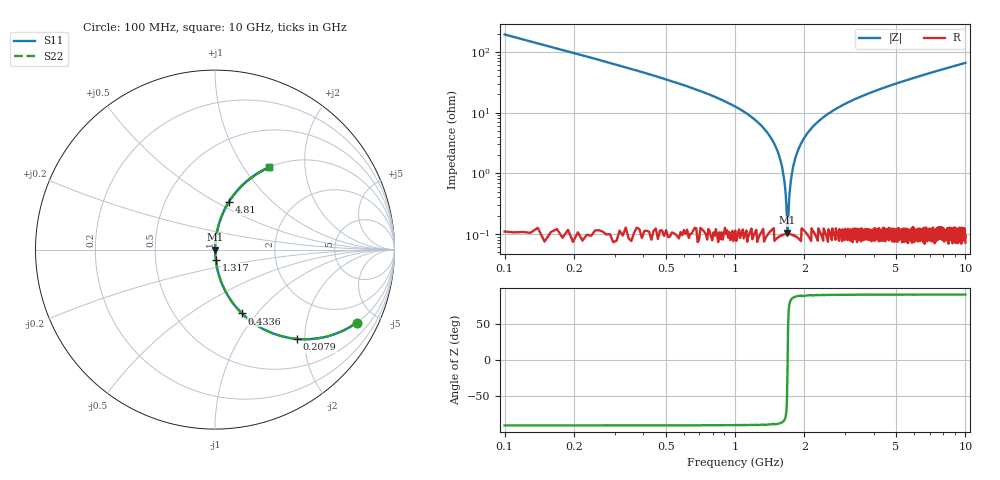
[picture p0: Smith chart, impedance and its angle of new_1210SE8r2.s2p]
!	AVX	Thin	Film	Operation	Date:	April 2007
!	Description:	Accu-P®	"Series,"	Thin	"Film,"	"SMD,"	RF	Capacitor
!	Part	Number:	12101J8R2BBT
!	100	MHz	-	5.05	GHz
!	Serial	Measurements
#	MHZ	S	MA	R	50
!	S11	S21	S12	S22
!	dB	Phase	dB	Phase	dB	Phase	dB	Phase
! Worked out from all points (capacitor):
!   1010 points, 100 MHz to 10 GHz, reference 50 ohm
!   read as one part in series: C = 8.2 pF near 149.1 MHz
!   lowest |Z| = 105 mohm at 1.689 GHz (marker M1)
!   series resonance near 1.692 GHz, so ESL is about 1.1 nH
!   S11 on the Smith chart (normalised r, x): 100 MHz: 1.00, -3.87; 207.9 MHz: 1.00, -1.84; 433.6 MHz: 1.00, -0.84; 1.317 GHz: 1.00, -0.12; 4.81 GHz: 1.00, +0.57; 10 GHz: 1.00, +1.32
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100  0.888 -27.3  0.459 62.6  0.459 62.6  0.888 -27.3
207.929  0.676 -47.4  0.736 42.6  0.736 42.6  0.676 -47.4
433.598  0.386 -67.2  0.922 22.7  0.922 22.7  0.386 -67.2
737.76  0.208 -77.7  0.977 12.0  0.977 12.0  0.208 -77.7
1316.65  0.058 -85.7  0.997 3.3  0.997 3.3  0.058 -85.7
1463.826  0.033 -86.4  0.998 1.9  0.998 1.9  0.033 -86.4
1552.131  0.02 -86.0  0.999 1.1  0.999 1.1  0.02 -86.0
1611.001  0.011 -84.3  0.999 0.6  0.999 0.6  0.011 -84.3
1660.059  0.00446 -76.8  0.999 0.2  0.999 0.2  0.00446 -76.8
1689.495  0.00105 -17.5  0.999 0.0  0.999 0.0  0.00105 -17.5
1728.741  0.00505 78.3  0.999 -0.3  0.999 -0.3  0.00505 78.3
1758.176  0.00888 83.0  0.999 -0.5  0.999 -0.5  0.00888 83.0
1817.047  0.016 85.6  0.999 -0.9  0.999 -0.9  0.016 85.6
1895.54  0.026 86.3  0.999 -1.5  0.999 -1.5  0.026 86.3
2189.891  0.06 85.6  0.997 -3.4  0.997 -3.4  0.06 85.6
2670.664  0.108 83.3  0.993 -6.2  0.993 -6.2  0.108 83.3
3406.541  0.171 79.8  0.984 -9.9  0.984 -9.9  0.171 79.8
4809.613  0.275 73.9  0.961 -15.9  0.961 -15.9  0.275 73.9
5054.906  0.291 72.9  0.956 -16.9  0.956 -16.9  0.291 72.9
6703.271  0.391 66.8  0.919 -23.0  0.919 -23.0  0.391 66.8
8351.635  0.477 61.4  0.878 -28.5  0.878 -28.5  0.477 61.4
10000  0.55 56.6  0.835 -33.3  0.835 -33.3  0.55 56.6
